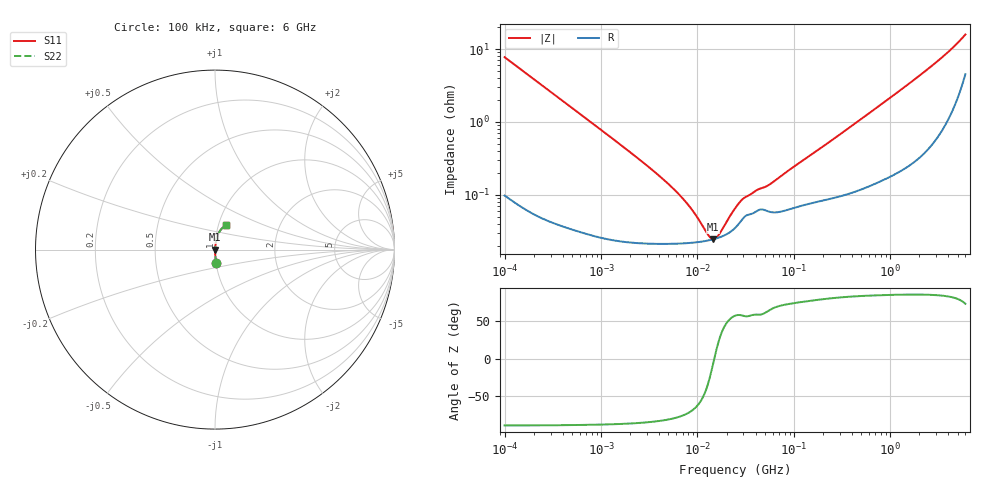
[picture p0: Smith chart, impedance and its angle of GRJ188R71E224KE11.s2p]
!Murata Part Number: GRJ188R71E224KE11
!These Parameters are Measured in Series Mode Connection
!Data Generated on Jun 19, 2026
!  o--ll--o
!Port1  Port2
!  o------o
!Operation Temp=25[degC], DC Bias Voltage=0[V]
!Freq. Start=100[kHz] Stop=6[GHz] 401[Steps]
# Hz S RI R 50
!Freq.(Hz) S11(Real) S11(Imag) S21(Real) S21(Imag) S12(Real) S12(Imag) S22(Real) S22(Imag)
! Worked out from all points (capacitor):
!   401 points, 100 kHz to 6 GHz, reference 50 ohm
!   read as one part in series: C = 206 nF near 105.7 kHz
!   lowest |Z| = 24.8 mohm at 14.52 MHz (marker M1)
!   series resonance near 14.93 MHz, so ESL is about 550 pH
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100000  0.0069 -0.0767  0.9931 0.0767  0.9931 0.0767  0.0069 -0.0767
222032  0.00173 -0.0349  0.9983 0.0349  0.9983 0.0349  0.00173 -0.0349
631452  0.000457 -0.0123  0.9995 0.0123  0.9995 0.0123  0.000457 -0.0123
2004685  0.000238 -0.00384  0.9998 0.00384  0.9998 0.00384  0.000238 -0.00384
3987316  0.000217 -0.00183  0.9998 0.00183  0.9998 0.00183  0.000217 -0.00183
5701257  0.000216 -0.00118  0.9998 0.00118  0.9998 0.00118  0.000216 -0.00118
7506273  0.000218 -0.000783  0.9998 0.000783  0.9998 0.000783  0.000218 -0.000783
9353785  0.000224 -0.000511  0.9998 0.000511  0.9998 0.000511  0.000224 -0.000511
1.301164e7  0.000238 -0.000146  0.9998 0.000146  0.9998 0.000146  0.000238 -0.000146
1.452491e7  0.000247 -2.95e-05  0.9998 2.95e-05  0.9998 2.95e-05  0.000247 -2.95e-05
1.534632e7  0.000252 2.88e-05  0.9997 -2.88e-05  0.9997 -2.88e-05  0.000252 2.88e-05
1.666634e7  0.000261 0.000117  0.9997 -0.000117  0.9997 -0.000117  0.000261 0.000117
2.517799e7  0.000366 0.000583  0.9996 -0.000583  0.9996 -0.000583  0.000366 0.000583
3.05238e7  0.000498 0.000765  0.9995 -0.000765  0.9995 -0.000765  0.000498 0.000765
4.130835e7  0.000603 0.000998  0.9994 -0.000998  0.9994 -0.000998  0.000603 0.000998
5.590324e7  0.00059 0.00126  0.9994 -0.00126  0.9994 -0.00126  0.00059 0.00126
1.546735e8  0.000787 0.00355  0.9992 -0.00355  0.9992 -0.00355  0.000787 0.00355
9.76689e8  0.00219 0.0209  0.9978 -0.0209  0.9978 -0.0209  0.00219 0.0209
2.052492e9  0.00524 0.0438  0.9948 -0.0438  0.9948 -0.0438  0.00524 0.0438
3.557862e9  0.0143 0.0778  0.9857 -0.0778  0.9857 -0.0778  0.0143 0.0778
4.814911e9  0.0307 0.1086  0.9693 -0.1086  0.9693 -0.1086  0.0307 0.1086
6e9  0.063 0.1359  0.937 -0.1359  0.937 -0.1359  0.063 0.1359
